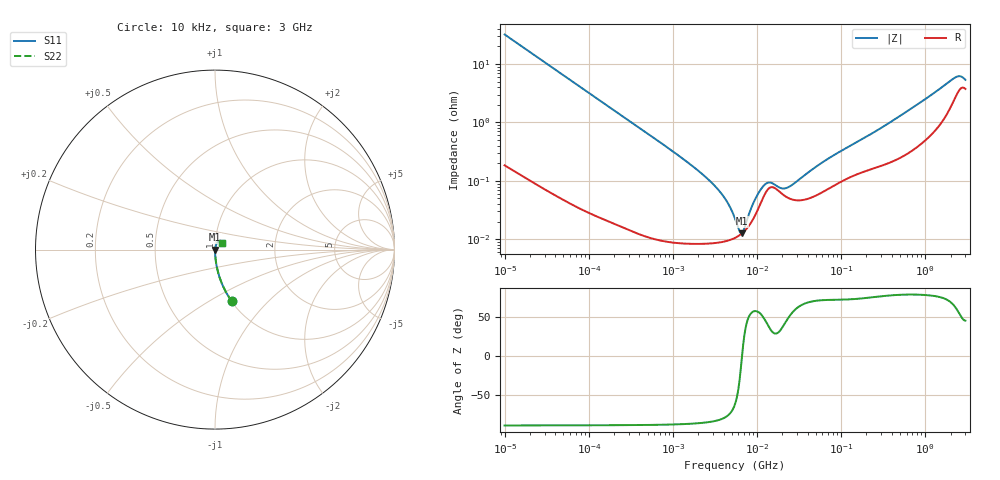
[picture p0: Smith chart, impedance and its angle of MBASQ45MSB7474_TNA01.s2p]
! MBASQ45MSB7474_TNA01  S-PARAMETER MODEL  ( Standard Model )
! Model Generated by TAIYO YUDEN Corporation (http://www.ty-top.com)
! Version 1.0
! TAIYO YUDEN Control No. 220601
! Copyright(c) 2013 TAIYO YUDEN CO.,LTD. All Rights Reserved.
! Product Description (link to TY-COMPAS)
! https://ds.yuden.co.jp/TYCOMPAS/or/detail?pn=MBASQ45MSB7474KTNA01&u=M
! Products Name : Multilayer Ceramic Capacitors
! Characteristics :
!  Capacitance : 0.47 [uF] , Rated Voltage : 250 [V] , TCC : X7R
!  Case Size : 4.5 x 3.2 / 0.177 x 0.126 [mm/inch] , Thickness : 2.5 / 0.098 [mm/inch]
!  (Conditions: Temperature = 25 [degC] , DC Bias Voltage = 0 [V])
! External Node Assignments :
!  1  o---| |---o  2
! GND o---------o GND
! Frequency Range : 10kHz  -  3GHz  [ 401 STEP ]
# MHZ S RI R 50
! Freq[MHz].  S11 Real  S11 Imag  S21 Real  S21 Imag  S12 Real  S12 Imag  S22 Real  S22 Imag
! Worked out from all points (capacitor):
!   401 points, 10 kHz to 3 GHz, reference 50 ohm
!   read as one part in series: C = 497 nF near 10.65 kHz
!   lowest |Z| = 12.6 mohm at 6.618 MHz (marker M1)
!   series resonance near 6.637 MHz, so ESL is about 1.2 nH
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0.01  0.0941 -0.2891  0.9059 0.2891  0.9059 0.2891  0.0941 -0.2891
0.026575  0.0151 -0.1188  0.9849 0.1188  0.9849 0.1188  0.0151 -0.1188
0.082683  0.00184 -0.0389  0.9982 0.0389  0.9982 0.0389  0.00184 -0.0389
0.683653  0.000119 -0.00471  0.9999 0.00471  0.9999 0.00471  0.000119 -0.00471
1.760434  8.63e-05 -0.00173  0.9999 0.00173  0.9999 0.00173  8.63e-05 -0.00173
3.008828  8.63e-05 -0.000875  0.9999 0.000875  0.9999 0.000875  8.63e-05 -0.000875
4.256163  9.29e-05 -0.000466  0.9999 0.000466  0.9999 0.000466  9.29e-05 -0.000466
5.477226  0.000106 -0.000201  0.9999 0.000201  0.9999 0.000201  0.000106 -0.000201
6.213436  0.000118 -6.96e-05  0.9999 6.96e-05  0.9999 6.96e-05  0.000118 -6.96e-05
6.617858  0.000126 -3.05e-06  0.9999 3.05e-06  0.9999 3.05e-06  0.000126 -3.05e-06
7.048603  0.000137 6.47e-05  0.9999 -6.47e-05  0.9999 -6.47e-05  0.000137 6.47e-05
9.361346  0.000246 0.000392  0.9998 -0.000392  0.9998 -0.000392  0.000246 0.000392
10.95979  0.000402 0.000567  0.9996 -0.000567  0.9996 -0.000567  0.000402 0.000567
12.43293  0.000596 0.000629  0.9994 -0.000629  0.9994 -0.000629  0.000596 0.000629
14.55585  0.000775 0.000516  0.9992 -0.000516  0.9992 -0.000516  0.000775 0.000516
19.33182  0.000618 0.000424  0.9994 -0.000424  0.9994 -0.000424  0.000618 0.000424
22.63272  0.000525 0.000548  0.9995 -0.000548  0.9995 -0.000548  0.000525 0.000548
45.28751  0.000526 0.00147  0.9995 -0.00147  0.9995 -0.00147  0.000526 0.00147
374.4521  0.00212 0.0096  0.9979 -0.0096  0.9979 -0.0096  0.00212 0.0096
2188.735  0.0257 0.0492  0.9743 -0.0492  0.9743 -0.0492  0.0257 0.0492
2562.461  0.0372 0.0465  0.9628 -0.0465  0.9628 -0.0465  0.0372 0.0465
3000  0.0373 0.0354  0.9627 -0.0354  0.9627 -0.0354  0.0373 0.0354
